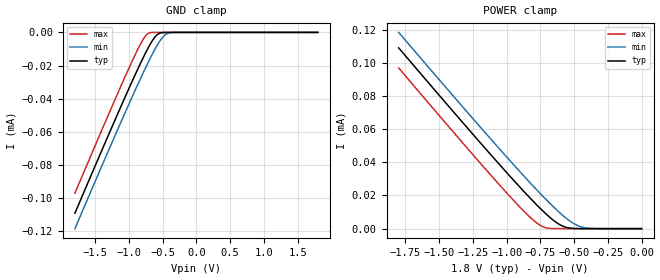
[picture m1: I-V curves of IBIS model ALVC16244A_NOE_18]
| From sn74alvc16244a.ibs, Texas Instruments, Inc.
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[Model]   ALVC16244A_NOE_18
Model_type  Input
Vinl=0.5775
Vinh=1.2675
| variable   typ   min   max
C_comp   0.71pF   0.50pF   0.81pF
[Temperature Range]   40   100   -40
| Ambient temperature   25   85   -40
[Voltage range]   1.8   1.65   1.95
[GND Clamp]
| ALVC16244A_NOE_18
|   Voltage   I(typ)   I(min)   I(max)
-1.8V     -109uA     -118.4uA   -96.92uA
-1.115V   -44.37uA   -53.81uA   -32.07uA
-930mV    -27.54uA   -36.91uA   -15.43uA
-810mV    -17.08uA   -26.26uA   -5.689uA
-760mV    -12.94uA   -21.94uA   -2.472uA
-720mV    -9.78uA    -18.56uA   -807.8nA
-615mV    -2.842uA   -10.21uA   -7.302nA
-550mV    -615.6nA   -5.713uA   -316pA
-465mV    -35.19nA   -1.565uA   -10.01pA
-405mV    -4.062nA   -366.8nA   -5.078pA
-310mV    -134.9pA   -22.79nA   -4.48pA
1.8V      3.324pA    181.7pA    2.876pA
[POWER Clamp]
| ALVC16244A_NOE_18
|   Voltage   I(typ)   I(min)   I(max)
-1.8V     109uA      118.4uA    96.92uA
-1.345V   65.82uA    75.25uA    53.56uA
-1.045V   37.94uA    47.37uA    25.67uA
-865mV    21.81uA    31.1uA     9.949uA
-760mV    12.94uA    21.94uA    2.472uA
-700mV    8.274uA    16.91uA    378.2nA
-645mV    4.523uA    12.49uA    31nA
-600mV    2.14uA     9.107uA    3.531nA
-545mV    530.2nA    5.404uA    249pA
-460mV    29.43nA    1.41uA     8.911pA
-360mV    801.6pA    101.5nA    4.682pA
-16.28fV  3.324pA    5.122pA    3.398pA
